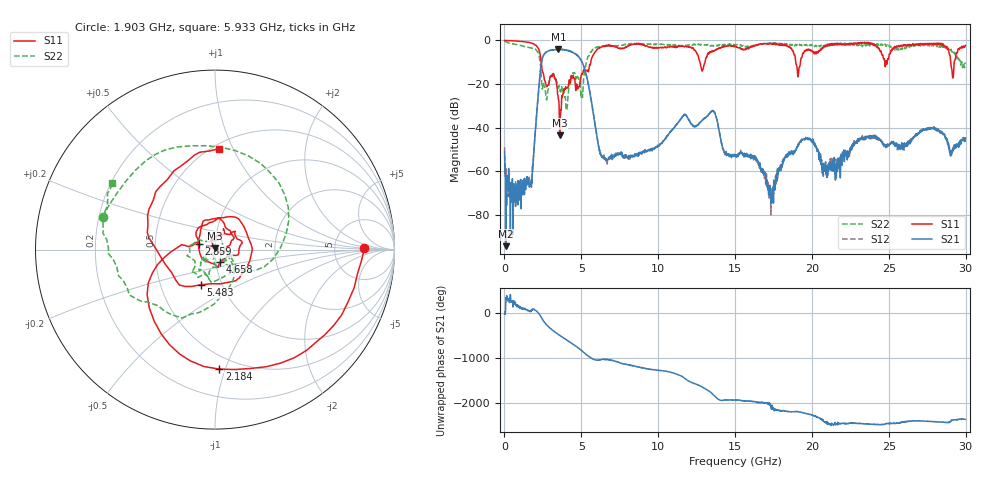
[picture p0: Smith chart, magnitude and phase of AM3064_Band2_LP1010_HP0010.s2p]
# Hz S DB R 50.0
!freq dBS11 angS11 dBS21 angS21 dBS12 angS12 dBS22 angS22
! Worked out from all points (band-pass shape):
!   1600 points, 10 MHz to 29.98 GHz, reference 50 ohm
!   highest |S21| = -4.00 dB at 3.515 GHz (marker M1); lowest = -94.2 dB at 84.97 MHz (marker M2)
!   |S21| within 3 dB of the highest: 2.537 GHz to 4.757 GHz (2.219 GHz wide, 60.9 % of centre)
!   lowest |S11| = -43.4 dB at 3.59 GHz (marker M3), VSWR 1.01, Z = 50.2 + j0.662 ohm
!   |S11| at or under -10 dB: 2.396 GHz to 5.618 GHz (3.221 GHz wide, 80.4 % of centre); 12.72 GHz to 13.05 GHz (329.5 MHz wide, 2.56 % of centre); 18.95 GHz to 19.25 GHz (303.9 MHz wide, 1.59 % of centre)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
!   |S22| runs from -31.7 to -0.3 dB; largest |S21 - S12| = 0.02
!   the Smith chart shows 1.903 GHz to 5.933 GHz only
!   S11 on the Smith chart (normalised r, x): 1.903 GHz: 11, +1; 2.184 GHz: 0.40, -0.95; 2.859 GHz: 0.83, +0.05; 4.658 GHz: 1.05, -0.15; 5.483 GHz: 0.79, -0.33; 5.933 GHz: 0.54, +0.88
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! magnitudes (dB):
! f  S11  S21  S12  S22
! 10 MHz  0.0  -51.3  -49.0  -0.3
! 84.97 MHz  0.0  -94.2  -60.0  -0.6
! 553.6 MHz  -0.2  -89.1  -73.3  -1.6
! 1.678 GHz  -1.1  -66.2  -65.9  -3.4
! 1.903 GHz  -1.6  -52.0  -51.1  -3.7
! 2.184 GHz  -3.5  -25.9  -25.9  -5.6
! 2.859 GHz  -20.5  -4.8  -4.8  -21.9
! 3.515 GHz  -27.3  -4.0  -4.2  -21.9
! 3.59 GHz  -43.4  -4.0  -4.1  -21.7
! 4.658 GHz  -22.4  -6.5  -6.3  -17.1
! 5.015 GHz  -15.3  -9.5  -9.4  -24.5
! 5.483 GHz  -13.5  -21.1  -21.0  -7.1
! 5.933 GHz  -5.0  -40.5  -40.6  -3.3
! 6.627 GHz  -2.5  -55.0  -54.9  -2.4
! 10 GHz  -3.4  -48.5  -47.9  -1.9
! 13.54 GHz  -5.2  -32.2  -32.0  -2.6
! 15 GHz  -2.7  -52.9  -53.1  -1.9
! 17.35 GHz  -1.3  -74.7  -70.9  -1.2
! 19.99 GHz  -4.6  -45.5  -46.0  -2.0
! 20.82 GHz  -2.7  -58.3  -59.0  -2.4
! 25 GHz  -8.0  -48.0  -48.7  -2.2
! 29.98 GHz  -2.4  -44.6  -46.1  -10.1
